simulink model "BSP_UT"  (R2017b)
settings: Solver=FixedStepDiscrete  StartTime=0.0  StopTime=10.0  FixedStep=0.01  RelTol=1e-3  EnableMultiTasking=on
undefined symbols (not defined in the file): ASWTYPE_FALSE, ASWTYPE_TRUE, CcBSP_CellVoltRngHiThrd_mV, CcBSP_CellVoltRngLowThrd_mV, CcBSP_ChrgMaxCellTempSaf_C, CcBSP_DCChrgNegTempHiThrd_C, CcBSP_DCChrgPosTempHiThrd_C, CcBSP_MaxCellTempSaf_C, CcBSP_MaxCellVoltSafDiff_mV, CcBSP_MinCellVoltSafDiff_mV, CcBSP_PackCurrSaf_A, Enum_CTCCtrCtlConnMode
libraries: AIWAYS_Powertrain_BMS_lib x14

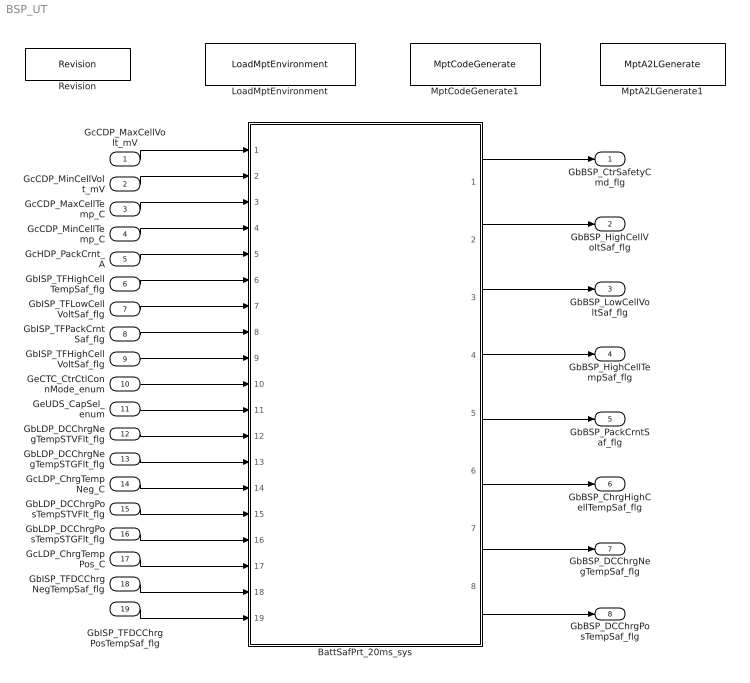
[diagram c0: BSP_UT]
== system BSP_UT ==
  GcCDP_MaxCellVolt_mV : Inport
  GcCDP_MinCellVolt_mV : Inport  Port=2
  GcCDP_MaxCellTemp_C : Inport  Port=3
  GcCDP_MinCellTemp_C : Inport  Port=4
  GcHDP_PackCrnt_A : Inport  Port=5
  GbISP_TFHighCellTempSaf_flg : Inport  Port=6
  GbISP_TFLowCellVoltSaf_flg : Inport  Port=7
  GbISP_TFPackCrntSaf_flg : Inport  Port=8
  GbISP_TFHighCellVoltSaf_flg : Inport  Port=9
  GeCTC_CtrCtlConnMode_enum : Inport  Port=10
  GeUDS_CapSel_enum : Inport  Port=11
  GbLDP_DCChrgNegTempSTVFlt_flg : Inport  Port=12
  GbLDP_DCChrgNegTempSTGFlt_flg : Inport  Port=13
  GcLDP_ChrgTempNeg_C : Inport  Port=14
  GbLDP_DCChrgPosTempSTVFlt_flg : Inport  Port=15
  GbLDP_DCChrgPosTempSTGFlt_flg : Inport  Port=16
  GcLDP_ChrgTempPos_C : Inport  Port=17
  GbISP_TFDCChrgNegTempSaf_flg : Inport  Port=18
  GbISP_TFDCChrgPosTempSaf_flg : Inport  Port=19
  BattSafPrt_20ms_sys : Subsystem
  LoadMptEnvironment : AIWAYS_Powertrain_BMS_lib/Config/LoadMptEnvironment  ProjectName=Comm  SuppierID=NewPlatformUAES
  MptA2LGenerate1 : AIWAYS_Powertrain_BMS_lib/Config/MptA2LGenerate  SystemSampleTime=-1
  MptCodeGenerate1 : AIWAYS_Powertrain_BMS_lib/Config/MptCodeGenerate  SystemSampleTime=-1
  Revision : AIWAYS_Powertrain_BMS_lib/Config/Revision  curVersion='M104C107'  newVersion='M104C107'
  GbBSP_CtrSafetyCmd_flg : Outport
  GbBSP_HighCellVoltSaf_flg : Outport  Port=2
  GbBSP_LowCellVoltSaf_flg : Outport  Port=3
  GbBSP_HighCellTempSaf_flg : Outport  Port=4
  GbBSP_PackCrntSaf_flg : Outport  Port=5
  GbBSP_ChrgHighCellTempSaf_flg : Outport  Port=6
  GbBSP_DCChrgNegTempSaf_flg : Outport  Port=7
  GbBSP_DCChrgPosTempSaf_flg : Outport  Port=8
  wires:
  GcLDP_ChrgTempNeg_C/1 -> BattSafPrt_20ms_sys/14(GcLDP_ChrgTempNeg_C)
  BattSafPrt_20ms_sys/7(GbBSP_DCChrgNegTempSaf_flg) -> GbBSP_DCChrgNegTempSaf_flg/1
  GbISP_TFHighCellVoltSaf_flg/1 -> BattSafPrt_20ms_sys/9(GbISP_TFHighCellVoltSaf_flg)
  GbISP_TFDCChrgPosTempSaf_flg/1 -> BattSafPrt_20ms_sys/19(GbISP_TFDCChrgPosTempSaf_flg)
  GbLDP_DCChrgPosTempSTVFlt_flg/1 -> BattSafPrt_20ms_sys/15(GbLDP_DCChrgPosTempSTVFlt_flg)
  GcHDP_PackCrnt_A/1 -> BattSafPrt_20ms_sys/5(GcHDP_PackCrnt_A)
  GcLDP_ChrgTempPos_C/1 -> BattSafPrt_20ms_sys/17(GcLDP_ChrgTempPos_C)
  GcCDP_MinCellVolt_mV/1 -> BattSafPrt_20ms_sys/2(GcCDP_MinCellVolt_mV)
  GbISP_TFHighCellTempSaf_flg/1 -> BattSafPrt_20ms_sys/6(GbISP_TFHighCellTempSaf_flg)
  GcCDP_MaxCellVolt_mV/1 -> BattSafPrt_20ms_sys/1(GcCDP_MaxCellVolt_mV)
  GbISP_TFDCChrgNegTempSaf_flg/1 -> BattSafPrt_20ms_sys/18(GbISP_TFDCChrgNegTempSaf_flg)
  GbLDP_DCChrgPosTempSTGFlt_flg/1 -> BattSafPrt_20ms_sys/16(GbLDP_DCChrgPosTempSTGFlt_flg)
  GcCDP_MaxCellTemp_C/1 -> BattSafPrt_20ms_sys/3(GcCDP_MaxCellTemp_C)
  BattSafPrt_20ms_sys/8(GbBSP_DCChrgPosTempSaf_flg) -> GbBSP_DCChrgPosTempSaf_flg/1
  BattSafPrt_20ms_sys/1(GbBSP_CtrSafetyCmd_flg) -> GbBSP_CtrSafetyCmd_flg/1
  GbLDP_DCChrgNegTempSTGFlt_flg/1 -> BattSafPrt_20ms_sys/13(GbLDP_DCChrgNegTempSTGFlt_flg)
  BattSafPrt_20ms_sys/2(GbBSP_HighCellVoltSaf_flg) -> GbBSP_HighCellVoltSaf_flg/1
  GcCDP_MinCellTemp_C/1 -> BattSafPrt_20ms_sys/4(GcCDP_MinCellTemp_C)
  BattSafPrt_20ms_sys/4(GbBSP_HighCellTempSaf_flg) -> GbBSP_HighCellTempSaf_flg/1
  BattSafPrt_20ms_sys/3(GbBSP_LowCellVoltSaf_flg) -> GbBSP_LowCellVoltSaf_flg/1
  BattSafPrt_20ms_sys/5(GbBSP_PackCrntSaf_flg) -> GbBSP_PackCrntSaf_flg/1
  GbLDP_DCChrgNegTempSTVFlt_flg/1 -> BattSafPrt_20ms_sys/12(GbLDP_DCChrgNegTempSTVFlt_flg)
  GbISP_TFPackCrntSaf_flg/1 -> BattSafPrt_20ms_sys/8(GbISP_TFPackCrntSaf_flg)
  GbISP_TFLowCellVoltSaf_flg/1 -> BattSafPrt_20ms_sys/7(GbISP_TFLowCellVoltSaf_flg)
  GeCTC_CtrCtlConnMode_enum/1 -> BattSafPrt_20ms_sys/10(GeCTC_CtrCtlConnMode_enum)
  BattSafPrt_20ms_sys/6(GbBSP_ChrgHighCellTempSaf_flg) -> GbBSP_ChrgHighCellTempSaf_flg/1
  GeUDS_CapSel_enum/1 -> BattSafPrt_20ms_sys/11(GeUDS_CapSel_enum)

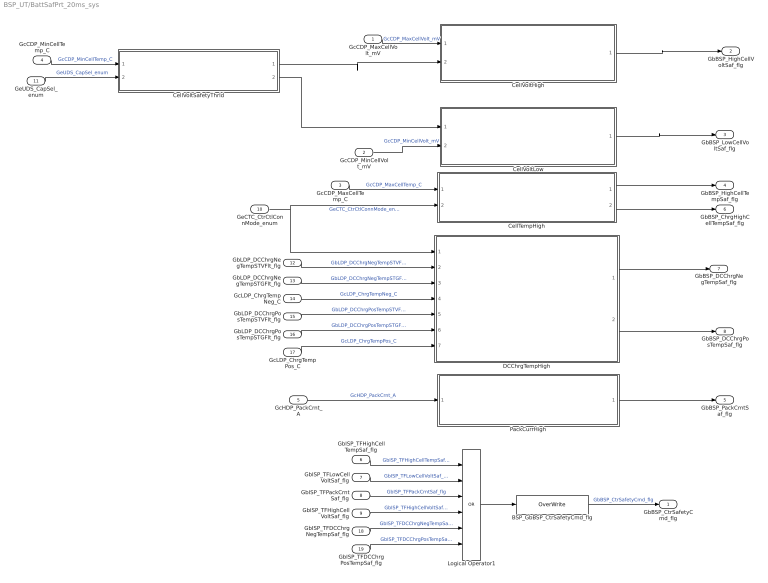
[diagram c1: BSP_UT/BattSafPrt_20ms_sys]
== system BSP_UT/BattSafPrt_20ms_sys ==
  GcCDP_MaxCellVolt_mV : Inport
  GcCDP_MinCellVolt_mV : Inport  Port=2
  GcCDP_MaxCellTemp_C : Inport  Port=3
  GcCDP_MinCellTemp_C : Inport  Port=4
  GcHDP_PackCrnt_A : Inport  Port=5
  GbISP_TFHighCellTempSaf_flg : Inport  Port=6
  GbISP_TFLowCellVoltSaf_flg : Inport  Port=7
  GbISP_TFPackCrntSaf_flg : Inport  Port=8
  GbISP_TFHighCellVoltSaf_flg : Inport  Port=9
  GeCTC_CtrCtlConnMode_enum : Inport  Port=10
  GeUDS_CapSel_enum : Inport  Port=11
  GbLDP_DCChrgNegTempSTVFlt_flg : Inport  Port=12
  GbLDP_DCChrgNegTempSTGFlt_flg : Inport  Port=13
  GcLDP_ChrgTempNeg_C : Inport  Port=14
  GbLDP_DCChrgPosTempSTVFlt_flg : Inport  Port=15
  GbLDP_DCChrgPosTempSTGFlt_flg : Inport  Port=16
  GcLDP_ChrgTempPos_C : Inport  Port=17
  GbISP_TFDCChrgNegTempSaf_flg : Inport  Port=18
  GbISP_TFDCChrgPosTempSaf_flg : Inport  Port=19
  BSP_GbBSP_CtrSafetyCmd_flg : AIWAYS_Powertrain_BMS_lib/Signals/OverWrite  OverWrite_Value=CbBSP_CtrSafetyCmdOvr_flg  OverWrite_flag=CbBSP_CtrSafetyCmdOvrSwt_flg
  CellTempHigh : Subsystem
  CellVoltHigh : Subsystem
  CellVoltLow : Subsystem
  CellVoltSafetyThrld : Subsystem
  DCChrgTempHigh : Subsystem
  Logical Operator1 : Logic  Operator=OR  Inputs=6  AllPortsSameDT=off  OutDataTypeStr=boolean
  PackCurrHigh : Subsystem
  GbBSP_CtrSafetyCmd_flg : Outport
  GbBSP_HighCellVoltSaf_flg : Outport  Port=2
  GbBSP_LowCellVoltSaf_flg : Outport  Port=3
  GbBSP_HighCellTempSaf_flg : Outport  Port=4
  GbBSP_PackCrntSaf_flg : Outport  Port=5
  GbBSP_ChrgHighCellTempSaf_flg : Outport  Port=6
  GbBSP_DCChrgNegTempSaf_flg : Outport  Port=7
  GbBSP_DCChrgPosTempSaf_flg : Outport  Port=8
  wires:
  GcCDP_MinCellTemp_C/1 -> CellVoltSafetyThrld/1(GcCDP_MinCellTemp_C)  "GcCDP_MinCellTemp_C"
  GcCDP_MaxCellVolt_mV/1 -> CellVoltHigh/1(GcCDP_MaxCellVolt_mV)  "GcCDP_MaxCellVolt_mV"
  CellVoltSafetyThrld/1(LcBSP_MaxCellVoltSafetyThrld_mV) -> CellVoltHigh/2(LcBSP_MaxCellVoltSafetyThrld_mV)
  CellVoltSafetyThrld/2(LcBSP_MinCellVoltSafetyThrld_mV) -> CellVoltLow/1(LcBSP_MinCellVoltSafetyThrld_mV)
  GcCDP_MinCellVolt_mV/1 -> CellVoltLow/2(GcCDP_MinCellVolt_mV)  "GcCDP_MinCellVolt_mV"
  GcCDP_MaxCellTemp_C/1 -> CellTempHigh/1(GcCDP_MaxCellTemp_C)  "GcCDP_MaxCellTemp_C"
  GcHDP_PackCrnt_A/1 -> PackCurrHigh/1(GcHDP_PackCrnt_A)  "GcHDP_PackCrnt_A"
  CellVoltHigh/1(GbBSP_HighCellVoltSaf_flg) -> GbBSP_HighCellVoltSaf_flg/1
  CellVoltLow/1(GbBSP_LowCellVoltSaf_flg) -> GbBSP_LowCellVoltSaf_flg/1
  CellTempHigh/1(GbBSP_HighCellTempSaf_flg) -> GbBSP_HighCellTempSaf_flg/1
  PackCurrHigh/1(GbBSP_PackCrntSaf_flg) -> GbBSP_PackCrntSaf_flg/1
  Logical Operator1/1 -> BSP_GbBSP_CtrSafetyCmd_flg/1
  BSP_GbBSP_CtrSafetyCmd_flg/1 -> GbBSP_CtrSafetyCmd_flg/1  "GbBSP_CtrSafetyCmd_flg"
  GbISP_TFHighCellTempSaf_flg/1 -> Logical Operator1/1  "GbISP_TFHighCellTempSaf_flg"
  GbISP_TFLowCellVoltSaf_flg/1 -> Logical Operator1/2  "GbISP_TFLowCellVoltSaf_flg"
  GbISP_TFPackCrntSaf_flg/1 -> Logical Operator1/3  "GbISP_TFPackCrntSaf_flg"
  GbISP_TFHighCellVoltSaf_flg/1 -> Logical Operator1/4  "GbISP_TFHighCellVoltSaf_flg"
  GeCTC_CtrCtlConnMode_enum/1 -> DCChrgTempHigh/1(GeCTC_CtrCtlConnMode_enum), CellTempHigh/2(GeCTC_CtrCtlConnMode_enum)  "GeCTC_CtrCtlConnMode_enum"
  CellTempHigh/2(GbBSP_ChrgHighCellTempSaf_flg) -> GbBSP_ChrgHighCellTempSaf_flg/1
  GeUDS_CapSel_enum/1 -> CellVoltSafetyThrld/2(GeUDS_CapSel_enum)  "GeUDS_CapSel_enum"
  GbLDP_DCChrgNegTempSTVFlt_flg/1 -> DCChrgTempHigh/2(GbLDP_DCChrgNegTempSTVFlt_flg)  "GbLDP_DCChrgNegTempSTVFlt_flg"
  GbLDP_DCChrgNegTempSTGFlt_flg/1 -> DCChrgTempHigh/3(GbLDP_DCChrgNegTempSTGFlt_flg)  "GbLDP_DCChrgNegTempSTGFlt_flg"
  GcLDP_ChrgTempNeg_C/1 -> DCChrgTempHigh/4(GcLDP_ChrgTempNeg_C)  "GcLDP_ChrgTempNeg_C"
  GbLDP_DCChrgPosTempSTVFlt_flg/1 -> DCChrgTempHigh/5(GbLDP_DCChrgPosTempSTVFlt_flg)  "GbLDP_DCChrgPosTempSTVFlt_flg"
  GbLDP_DCChrgPosTempSTGFlt_flg/1 -> DCChrgTempHigh/6(GbLDP_DCChrgPosTempSTGFlt_flg)  "GbLDP_DCChrgPosTempSTGFlt_flg"
  GcLDP_ChrgTempPos_C/1 -> DCChrgTempHigh/7(GcLDP_ChrgTempPos_C)  "GcLDP_ChrgTempPos_C"
  DCChrgTempHigh/2(GbBSP_DCChrgPosTempSaf_flg) -> GbBSP_DCChrgPosTempSaf_flg/1
  DCChrgTempHigh/1(GbBSP_DCChrgNegTempSaf_flg) -> GbBSP_DCChrgNegTempSaf_flg/1
  GbISP_TFDCChrgNegTempSaf_flg/1 -> Logical Operator1/5  "GbISP_TFDCChrgNegTempSaf_flg"
  GbISP_TFDCChrgPosTempSaf_flg/1 -> Logical Operator1/6  "GbISP_TFDCChrgPosTempSaf_flg"

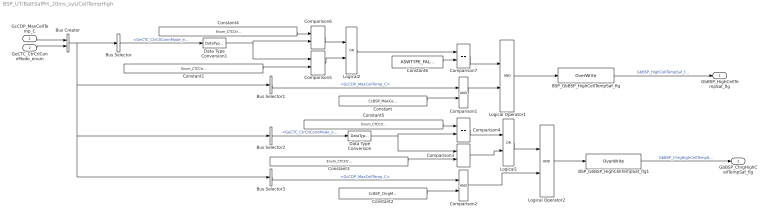
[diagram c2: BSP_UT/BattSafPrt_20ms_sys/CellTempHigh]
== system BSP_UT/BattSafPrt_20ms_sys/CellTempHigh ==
  GcCDP_MaxCellTemp_C : Inport
  GeCTC_CtrCtlConnMode_enum : Inport  Port=2
  BSP_GbBSP_HighCellTempSaf_flg : AIWAYS_Powertrain_BMS_lib/Signals/OverWrite  OverWrite_Value=CbBSP_HighCellTempSafOvr_flg  OverWrite_flag=CbBSP_HighCellTempSafOvrSwt_flg
  BSP_GbBSP_HighCellTempSaf_flg1 : AIWAYS_Powertrain_BMS_lib/Signals/OverWrite  OverWrite_Value=CbBSP_ChrgHighCellTempSafOvr_flg  OverWrite_flag=CbBSP_ChrgHighCellTempSafOvrSwt_flg
  Bus Creator : BusCreator  Inputs=2
  Bus Selector : BusSelector  OutputSignals=GeCTC_CtrCtlConnMode_enum
  Bus Selector1 : BusSelector  OutputSignals=GcCDP_MaxCellTemp_C
  Bus Selector2 : BusSelector  OutputSignals=GeCTC_CtrCtlConnMode_enum
  Bus Selector3 : BusSelector  OutputSignals=GcCDP_MaxCellTemp_C
  Comparison1 : RelationalOperator  OutDataTypeStr=boolean
  Comparison2 : RelationalOperator  OutDataTypeStr=boolean
  Comparison{3..7} (5 alike) : RelationalOperator  Operator===  OutDataTypeStr=boolean
  Constant : Constant  Value=CcBSP_MaxCellTempSaf_C
  Constant1 : Constant  Value=Enum_CTCCtrCtlConnMode.Enum_CTCCtrCtlConnMode_ACChrg
  Constant2 : Constant  Value=CcBSP_ChrgMaxCellTempSaf_C
  Constant3 : Constant  Value=Enum_CTCCtrCtlConnMode.Enum_CTCCtrCtlConnMode_ACChrg
  Constant4 : Constant  Value=Enum_CTCCtrCtlConnMode.Enum_CTCCtrCtlConnMode_DCChrg
  Constant5 : Constant  Value=Enum_CTCCtrCtlConnMode.Enum_CTCCtrCtlConnMode_DCChrg
  Constant6 : Constant  Value=ASWTYPE_FALSE
  Data Type Conversion : DataTypeConversion
  Data Type Conversion1 : DataTypeConversion
  Logical Operator1 : Logic  AllPortsSameDT=off  OutDataTypeStr=boolean
  Logical Operator2 : Logic  AllPortsSameDT=off  OutDataTypeStr=boolean
  Logical1 : Logic  Operator=OR  OutDataTypeStr=boolean
  Logical2 : Logic  Operator=OR  OutDataTypeStr=boolean
  GbBSP_HighCellTempSaf_flg : Outport
  GbBSP_ChrgHighCellTempSaf_flg : Outport  Port=2
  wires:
  Constant/1 -> Comparison1/2
  BSP_GbBSP_HighCellTempSaf_flg/1 -> GbBSP_HighCellTempSaf_flg/1  "GbBSP_HighCellTempSaf_flg"
  Comparison1/1 -> Logical Operator1/2
  Logical Operator1/1 -> BSP_GbBSP_HighCellTempSaf_flg/1
  Bus Selector3/1 -> Comparison2/1  "<GcCDP_MaxCellTemp_C>"
  Constant2/1 -> Comparison2/2
  Comparison2/1 -> Logical Operator2/2
  Logical Operator2/1 -> BSP_GbBSP_HighCellTempSaf_flg1/1
  Logical1/1 -> Logical Operator2/1
  Data Type Conversion/1 -> Comparison3/1, Comparison4/2
  BSP_GbBSP_HighCellTempSaf_flg1/1 -> GbBSP_ChrgHighCellTempSaf_flg/1  "GbBSP_ChrgHighCellTempSaf_flg"
  GeCTC_CtrCtlConnMode_enum/1 -> Bus Creator/2
  Constant3/1 -> Comparison3/2
  Comparison4/1 -> Logical1/1
  Constant5/1 -> Comparison4/1
  Comparison3/1 -> Logical1/2
  GcCDP_MaxCellTemp_C/1 -> Bus Creator/1
  Bus Creator/1 -> Bus Selector3/1, Bus Selector2/1, Bus Selector1/1, Bus Selector/1
  Comparison5/1 -> Logical2/2
  Constant4/1 -> Comparison6/1
  Comparison6/1 -> Logical2/1
  Constant1/1 -> Comparison5/2
  Data Type Conversion1/1 -> Comparison6/2, Comparison5/1
  Logical2/1 -> Comparison7/1
  Bus Selector/1 -> Data Type Conversion1/1  "<GeCTC_CtrCtlConnMode_enum>"
  Constant6/1 -> Comparison7/2
  Comparison7/1 -> Logical Operator1/1
  Bus Selector1/1 -> Comparison1/1  "<GcCDP_MaxCellTemp_C>"
  Bus Selector2/1 -> Data Type Conversion/1  "<GeCTC_CtrCtlConnMode_enum>"

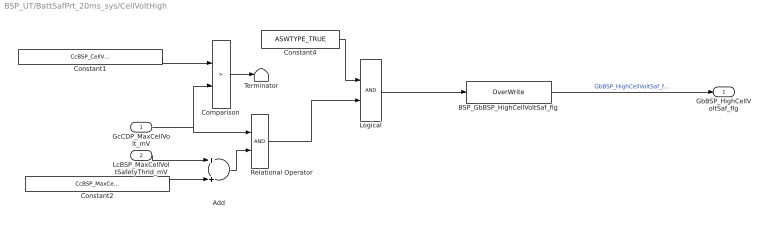
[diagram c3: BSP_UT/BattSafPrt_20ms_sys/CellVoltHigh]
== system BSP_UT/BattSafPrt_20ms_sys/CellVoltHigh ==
  GcCDP_MaxCellVolt_mV : Inport
  LcBSP_MaxCellVoltSafetyThrld_mV : Inport  Port=2
  Add : Sum
  BSP_GbBSP_HighCellVoltSaf_flg : AIWAYS_Powertrain_BMS_lib/Signals/OverWrite  OverWrite_Value=CbBSP_HighCellVoltSafOvr_flg  OverWrite_flag=CbBSP_HighCellVoltSafOvrSwt_flg
  Comparison : RelationalOperator  Operator=>  OutDataTypeStr=boolean
  Constant1 : Constant  Value=CcBSP_CellVoltRngHiThrd_mV
  Constant2 : Constant  Value=CcBSP_MaxCellVoltSafDiff_mV
  Constant4 : Constant  Value=ASWTYPE_TRUE
  Logical : Logic  OutDataTypeStr=boolean
  Relational Operator : RelationalOperator  OutDataTypeStr=boolean
  Terminator : Terminator
  GbBSP_HighCellVoltSaf_flg : Outport
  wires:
  GcCDP_MaxCellVolt_mV/1 -> Comparison/2, Relational Operator/1
  BSP_GbBSP_HighCellVoltSaf_flg/1 -> GbBSP_HighCellVoltSaf_flg/1  "GbBSP_HighCellVoltSaf_flg"
  Logical/1 -> BSP_GbBSP_HighCellVoltSaf_flg/1
  Add/1 -> Relational Operator/2
  LcBSP_MaxCellVoltSafetyThrld_mV/1 -> Add/1
  Constant2/1 -> Add/2
  Relational Operator/1 -> Logical/2
  Constant1/1 -> Comparison/1
  Comparison/1 -> Terminator/1
  Constant4/1 -> Logical/1

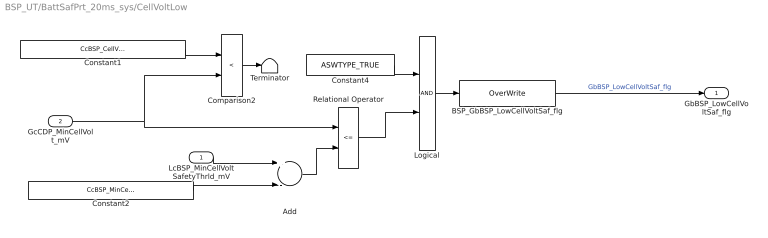
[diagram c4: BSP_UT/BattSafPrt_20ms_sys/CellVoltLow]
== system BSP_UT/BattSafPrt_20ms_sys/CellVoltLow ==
  LcBSP_MinCellVoltSafetyThrld_mV : Inport
  GcCDP_MinCellVolt_mV : Inport  Port=2
  Add : Sum  Inputs=+-
  BSP_GbBSP_LowCellVoltSaf_flg : AIWAYS_Powertrain_BMS_lib/Signals/OverWrite  OverWrite_Value=CbBSP_LowCellVoltSafOvr_flg  OverWrite_flag=CbBSP_LowCellVoltSafOvrSwt_flg
  Comparison2 : RelationalOperator  Operator=<  OutDataTypeStr=boolean
  Constant1 : Constant  Value=CcBSP_CellVoltRngLowThrd_mV
  Constant2 : Constant  Value=CcBSP_MinCellVoltSafDiff_mV
  Constant4 : Constant  Value=ASWTYPE_TRUE
  Logical : Logic  OutDataTypeStr=boolean
  Relational Operator : RelationalOperator  Operator=<=  OutDataTypeStr=boolean
  Terminator : Terminator
  GbBSP_LowCellVoltSaf_flg : Outport
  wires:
  GcCDP_MinCellVolt_mV/1 -> Relational Operator/1, Comparison2/2
  BSP_GbBSP_LowCellVoltSaf_flg/1 -> GbBSP_LowCellVoltSaf_flg/1  "GbBSP_LowCellVoltSaf_flg"
  Relational Operator/1 -> Logical/2
  Add/1 -> Relational Operator/2
  LcBSP_MinCellVoltSafetyThrld_mV/1 -> Add/1
  Constant2/1 -> Add/2
  Constant1/1 -> Comparison2/1
  Comparison2/1 -> Terminator/1
  Logical/1 -> BSP_GbBSP_LowCellVoltSaf_flg/1
  Constant4/1 -> Logical/1

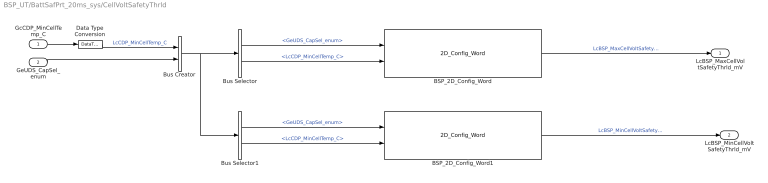
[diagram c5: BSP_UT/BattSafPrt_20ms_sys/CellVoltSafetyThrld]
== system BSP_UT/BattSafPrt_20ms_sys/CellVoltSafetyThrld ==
  GcCDP_MinCellTemp_C : Inport
  GeUDS_CapSel_enum : Inport  Port=2
  BSP_2D_Config_Word : AIWAYS_Powertrain_BMS_lib/Signals/2D_Config_Word  Default_Cal_Breakpoint1_Name=CaBSP_MaxCellVoltSafTempTab_C  Default_Cal_Table1_Name=CaBSP_CATL177MaxCellVoltSafVoltTab_mV  CATL153Ah_Cal_Breakpoint1_Name=CaBSP_MaxCellVoltSafTempTab_C  CATL153Ah_Cal_Table1_Name=CaBSP_CATL177MaxCellVoltSafVoltTab_mV  CATL180Ah_Cal_Breakpoint1_Name=CaBSP_MaxCellVoltSafTempTab_C  CATL180Ah_Cal_Table1_Name=CaBSP_CATL177MaxCellVoltSafVoltTab_mV  CATL177Ah_Cal_Breakpoint1_Name=CaBSP_MaxCellVoltSafTempTab_C  CATL177Ah_Cal_Table1_Name=CaBSP_CATL177MaxCellVoltSafVoltTab_mV  CATL203Ah_Cal_Breakpoint1_Name=CaBSP_MaxCellVoltSafTempTab_C  CATL203Ah_Cal_Table1_Name=CaBSP_CATL203MaxCellVoltSafVoltTab_mV  CATL51Ah_Cal_Breakpoint1_Name=CaBSP_MaxCellVoltSafTempTab_C  CATL51Ah_Cal_Table1_Name=CaBSP_CATL177MaxCellVoltSafVoltTab_mV  CATL132Ah_Cal_Breakpoint1_Name=CaBSP_MaxCellVoltSafTempTab_C  CATL132Ah_Cal_Table1_Name=CaBSP_CATL177MaxCellVoltSafVoltTab_mV  XWD75Ah_Cal_Breakpoint1_Name=CaBSP_MaxCellVoltSafTempTab_C  XWD75Ah_Cal_Table1_Name=CaBSP_XWD75MaxCellVoltSafVoltTab_mV  TFE177Ah_Cal_Breakpoint1_Name=CaBSP_MaxCellVoltSafTempTab_C  TFE177Ah_Cal_Table1_Name=CaBSP_TFE177MaxCellVoltSafVoltTab_mV  CATLCTP248Ah_Cal_Breakpoint1_Name=CaBSP_MaxCellVoltSafTempTab_C  CATLCTP248Ah_Cal_Table1_Name=CaBSP_CATL177MaxCellVoltSafVoltTab_mV
  BSP_2D_Config_Word1 : AIWAYS_Powertrain_BMS_lib/Signals/2D_Config_Word  Default_Cal_Breakpoint1_Name=CaBSP_MinCellVoltSafTempTab_C  Default_Cal_Table1_Name=CaBSP_CATL177MinCellVoltSafVoltTab_mV  CATL153Ah_Cal_Breakpoint1_Name=CaBSP_MinCellVoltSafTempTab_C  CATL153Ah_Cal_Table1_Name=CaBSP_CATL177MinCellVoltSafVoltTab_mV  CATL180Ah_Cal_Breakpoint1_Name=CaBSP_MinCellVoltSafTempTab_C  CATL180Ah_Cal_Table1_Name=CaBSP_CATL177MinCellVoltSafVoltTab_mV  CATL177Ah_Cal_Breakpoint1_Name=CaBSP_MinCellVoltSafTempTab_C  CATL177Ah_Cal_Table1_Name=CaBSP_CATL177MinCellVoltSafVoltTab_mV  CATL203Ah_Cal_Breakpoint1_Name=CaBSP_MinCellVoltSafTempTab_C  CATL203Ah_Cal_Table1_Name=CaBSP_CATL203MinCellVoltSafVoltTab_mV  CATL51Ah_Cal_Breakpoint1_Name=CaBSP_MinCellVoltSafTempTab_C  CATL51Ah_Cal_Table1_Name=CaBSP_CATL177MinCellVoltSafVoltTab_mV  CATL132Ah_Cal_Breakpoint1_Name=CaBSP_MinCellVoltSafTempTab_C  CATL132Ah_Cal_Table1_Name=CaBSP_CATL177MinCellVoltSafVoltTab_mV  XWD75Ah_Cal_Breakpoint1_Name=CaBSP_MinCellVoltSafTempTab_C  XWD75Ah_Cal_Table1_Name=CaBSP_XWD75MinCellVoltSafVoltTab_mV  TFE177Ah_Cal_Breakpoint1_Name=CaBSP_MinCellVoltSafTempTab_C  TFE177Ah_Cal_Table1_Name=CaBSP_TFE177MinCellVoltSafVoltTab_mV  CATLCTP248Ah_Cal_Breakpoint1_Name=CaBSP_MinCellVoltSafTempTab_C  CATLCTP248Ah_Cal_Table1_Name=CaBSP_CATL177MinCellVoltSafVoltTab_mV
  Bus Creator : BusCreator  Inputs=2
  Bus Selector : BusSelector  OutputSignals=GeUDS_CapSel_enum,LcCDP_MinCellTemp_C
  Bus Selector1 : BusSelector  OutputSignals=GeUDS_CapSel_enum,LcCDP_MinCellTemp_C
  Data Type Conversion : DataTypeConversion  OutDataTypeStr=fixdt(0,8,1,-40)
  LcBSP_MaxCellVoltSafetyThrld_mV : Outport
  LcBSP_MinCellVoltSafetyThrld_mV : Outport  Port=2
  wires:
  GcCDP_MinCellTemp_C/1 -> Data Type Conversion/1
  BSP_2D_Config_Word/1 -> LcBSP_MaxCellVoltSafetyThrld_mV/1  "LcBSP_MaxCellVoltSafetyThrld_mV"
  BSP_2D_Config_Word1/1 -> LcBSP_MinCellVoltSafetyThrld_mV/1  "LcBSP_MinCellVoltSafetyThrld_mV"
  Data Type Conversion/1 -> Bus Creator/1  "LcCDP_MinCellTemp_C"
  GeUDS_CapSel_enum/1 -> Bus Creator/2
  Bus Creator/1 -> Bus Selector1/1, Bus Selector/1
  Bus Selector/1 -> BSP_2D_Config_Word/1  "<GeUDS_CapSel_enum>"
  Bus Selector/2 -> BSP_2D_Config_Word/2  "<LcCDP_MinCellTemp_C>"
  Bus Selector1/1 -> BSP_2D_Config_Word1/1  "<GeUDS_CapSel_enum>"
  Bus Selector1/2 -> BSP_2D_Config_Word1/2  "<LcCDP_MinCellTemp_C>"

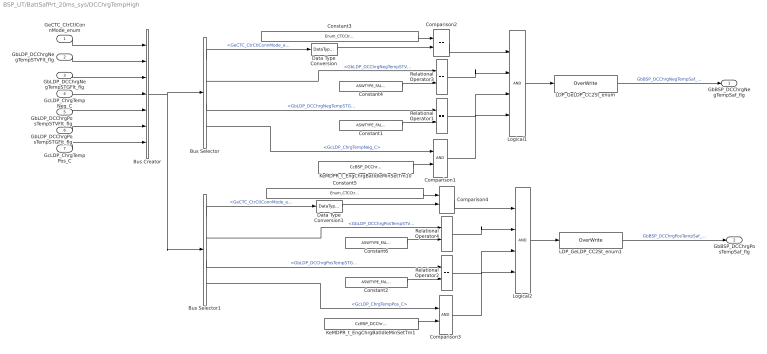
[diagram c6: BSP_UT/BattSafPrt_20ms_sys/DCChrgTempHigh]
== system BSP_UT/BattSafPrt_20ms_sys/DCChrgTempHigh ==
  GeCTC_CtrCtlConnMode_enum : Inport
  GbLDP_DCChrgNegTempSTVFlt_flg : Inport  Port=2
  GbLDP_DCChrgNegTempSTGFlt_flg : Inport  Port=3
  GcLDP_ChrgTempNeg_C : Inport  Port=4
  GbLDP_DCChrgPosTempSTVFlt_flg : Inport  Port=5
  GbLDP_DCChrgPosTempSTGFlt_flg : Inport  Port=6
  GcLDP_ChrgTempPos_C : Inport  Port=7
  Bus Creator : BusCreator  Inputs=7
  Bus Selector : BusSelector  OutputSignals=GeCTC_CtrCtlConnMode_enum,GbLDP_DCChrgNegTempSTVFlt_flg,GbLDP_DCChrgNegTempSTGFlt_flg,GcLDP_ChrgTempNeg_C
  Bus Selector1 : BusSelector  OutputSignals=GeCTC_CtrCtlConnMode_enum,GbLDP_DCChrgPosTempSTVFlt_flg,GbLDP_DCChrgPosTempSTGFlt_flg,GcLDP_ChrgTempPos_C
  Comparison1 : RelationalOperator  OutDataTypeStr=boolean
  Comparison2 : RelationalOperator  Operator===  OutDataTypeStr=boolean
  Comparison3 : RelationalOperator  OutDataTypeStr=boolean
  Comparison4 : RelationalOperator  Operator===  OutDataTypeStr=boolean
  Constant{1..2,4,6} (4 alike) : Constant  Value=ASWTYPE_FALSE
  Constant3 : Constant  Value=Enum_CTCCtrCtlConnMode.Enum_CTCCtrCtlConnMode_DCChrg
  Constant5 : Constant  Value=Enum_CTCCtrCtlConnMode.Enum_CTCCtrCtlConnMode_DCChrg
  Data Type Conversion : DataTypeConversion
  Data Type Conversion1 : DataTypeConversion
  KeMDPR_t_EngChrgBatIdleMinSetTm1 : Constant  Value=CcBSP_DCChrgPosTempHiThrd_C
  KeMDPR_t_EngChrgBatIdleMinSetTm10 : Constant  Value=CcBSP_DCChrgNegTempHiThrd_C
  LDP_GeLDP_CC2St_enum : AIWAYS_Powertrain_BMS_lib/Signals/OverWrite  OverWrite_Value=CbBSP_DCChrgNegTempSafOvr_flg  OverWrite_flag=CbBSP_DCChrgNegTempSafOvrSwt_flg
  LDP_GeLDP_CC2St_enum1 : AIWAYS_Powertrain_BMS_lib/Signals/OverWrite  OverWrite_Value=CbBSP_DCChrgPosTempSafOvr_flg  OverWrite_flag=CbBSP_DCChrgPosTempSafOvrSwt_flg
  Logical1 : Logic  Inputs=4  OutDataTypeStr=boolean
  Logical2 : Logic  Inputs=4  OutDataTypeStr=boolean
  Relational Operator{1..4} (4 alike) : RelationalOperator  Operator===  OutDataTypeStr=boolean
  GbBSP_DCChrgNegTempSaf_flg : Outport
  GbBSP_DCChrgPosTempSaf_flg : Outport  Port=2
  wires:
  Comparison1/1 -> Logical1/4
  Relational Operator3/1 -> Logical1/2
  GcLDP_ChrgTempNeg_C/1 -> Bus Creator/4
  GbLDP_DCChrgNegTempSTGFlt_flg/1 -> Bus Creator/3
  GbLDP_DCChrgNegTempSTVFlt_flg/1 -> Bus Creator/2
  KeMDPR_t_EngChrgBatIdleMinSetTm10/1 -> Comparison1/2
  Constant1/1 -> Relational Operator1/2
  Relational Operator1/1 -> Logical1/3
  Constant3/1 -> Comparison2/1
  Comparison2/1 -> Logical1/1
  Data Type Conversion/1 -> Comparison2/2
  GeCTC_CtrCtlConnMode_enum/1 -> Bus Creator/1
  Constant4/1 -> Relational Operator3/2
  Logical1/1 -> LDP_GeLDP_CC2St_enum/1
  LDP_GeLDP_CC2St_enum/1 -> GbBSP_DCChrgNegTempSaf_flg/1  "GbBSP_DCChrgNegTempSaf_flg"
  LDP_GeLDP_CC2St_enum1/1 -> GbBSP_DCChrgPosTempSaf_flg/1  "GbBSP_DCChrgPosTempSaf_flg"
  Data Type Conversion1/1 -> Comparison4/2
  Constant6/1 -> Relational Operator4/2
  Relational Operator4/1 -> Logical2/2
  Relational Operator2/1 -> Logical2/3
  GbLDP_DCChrgPosTempSTVFlt_flg/1 -> Bus Creator/5
  GcLDP_ChrgTempPos_C/1 -> Bus Creator/7
  Constant5/1 -> Comparison4/1
  Comparison4/1 -> Logical2/1
  KeMDPR_t_EngChrgBatIdleMinSetTm1/1 -> Comparison3/2
  GbLDP_DCChrgPosTempSTGFlt_flg/1 -> Bus Creator/6
  Comparison3/1 -> Logical2/4
  Constant2/1 -> Relational Operator2/2
  Logical2/1 -> LDP_GeLDP_CC2St_enum1/1
  Bus Creator/1 -> Bus Selector1/1, Bus Selector/1
  Bus Selector/1 -> Data Type Conversion/1  "<GeCTC_CtrCtlConnMode_enum>"
  Bus Selector/2 -> Relational Operator3/1  "<GbLDP_DCChrgNegTempSTVFlt_flg>"
  Bus Selector/3 -> Relational Operator1/1  "<GbLDP_DCChrgNegTempSTGFlt_flg>"
  Bus Selector/4 -> Comparison1/1  "<GcLDP_ChrgTempNeg_C>"
  Bus Selector1/1 -> Data Type Conversion1/1  "<GeCTC_CtrCtlConnMode_enum>"
  Bus Selector1/2 -> Relational Operator4/1  "<GbLDP_DCChrgPosTempSTVFlt_flg>"
  Bus Selector1/3 -> Relational Operator2/1  "<GbLDP_DCChrgPosTempSTGFlt_flg>"
  Bus Selector1/4 -> Comparison3/1  "<GcLDP_ChrgTempPos_C>"

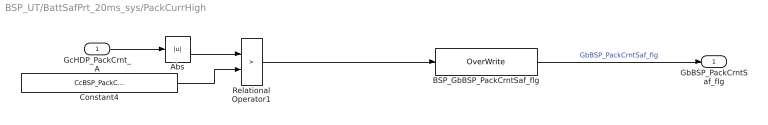
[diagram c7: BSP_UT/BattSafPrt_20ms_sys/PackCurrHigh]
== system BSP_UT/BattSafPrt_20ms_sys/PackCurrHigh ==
  GcHDP_PackCrnt_A : Inport
  Abs : Abs
  BSP_GbBSP_PackCrntSaf_flg : AIWAYS_Powertrain_BMS_lib/Signals/OverWrite  OverWrite_Value=CbBSP_PackCrntSafOvr_flg  OverWrite_flag=CbBSP_PackCrntSafOvrSwt_flg
  Constant4 : Constant  Value=CcBSP_PackCurrSaf_A
  Relational Operator1 : RelationalOperator  Operator=>  OutDataTypeStr=boolean
  GbBSP_PackCrntSaf_flg : Outport
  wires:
  Relational Operator1/1 -> BSP_GbBSP_PackCrntSaf_flg/1
  BSP_GbBSP_PackCrntSaf_flg/1 -> GbBSP_PackCrntSaf_flg/1  "GbBSP_PackCrntSaf_flg"
  Constant4/1 -> Relational Operator1/2
  GcHDP_PackCrnt_A/1 -> Abs/1
  Abs/1 -> Relational Operator1/1
